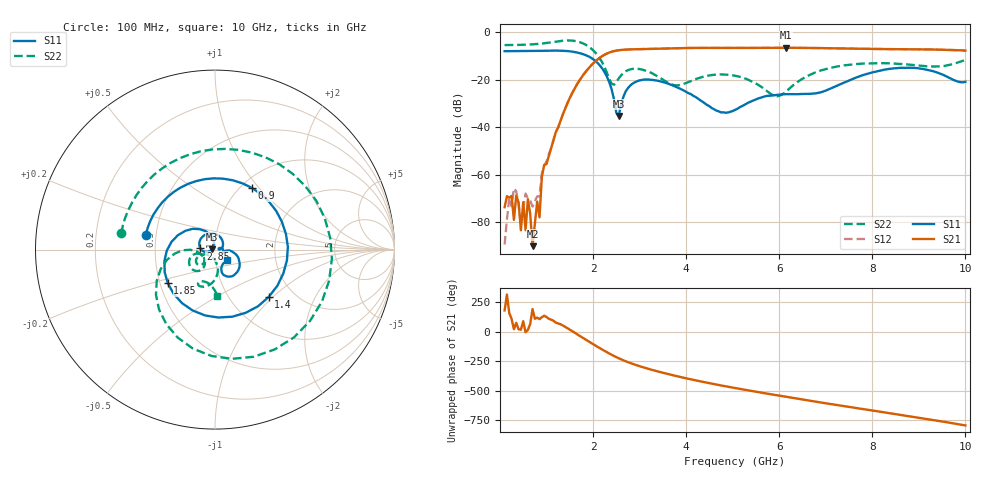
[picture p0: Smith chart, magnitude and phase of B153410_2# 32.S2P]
!  2-Port S-parameters saved by WinCal
! VAR MeasName=S-Parameters (CALIBRATED_DATA) read from VNA (N5245A)
! VAR MeasDate=2016-12-23 10:00:58
! VAR NAME=B153410_2# 32
! VAR FILENAME=B153410_2# 32.S2P
! VAR DATE=2016-12-23 10:00:58
! VAR PHYS_PORTS=1,2
# Hz S DB R 50
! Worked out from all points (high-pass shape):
!   199 points, 100 MHz to 10 GHz, reference 50 ohm
!   highest |S21| = -6.64 dB at 6.15 GHz (marker M1); lowest = -90.1 dB at 700 MHz (marker M2)
!   |S21| within 3 dB of the highest: 2.242 GHz to end of sweep
!   lowest |S11| = -35.4 dB at 2.55 GHz (marker M3), VSWR 1.03, Z = 48.3 + j0.252 ohm
!   |S11| at or under -10 dB: 1.871 GHz to end of sweep
!   |S22| runs from -27.1 to -3.6 dB; largest |S21 - S12| = 0.004
!   S11 on the Smith chart (normalised r, x): 100 MHz: 0.44, +0.08; 900 MHz: 1.12, +0.92; 1.4 GHz: 1.50, -0.94; 1.85 GHz: 0.55, -0.23; 2.85 GHz: 0.85, +0.01; 10 GHz: 1.13, -0.14
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1e8  -8.09 168.3  -73.70 179.7  -89.45 106.2  -5.52 170.2
2.5e8  -8.08 150.5  -68.95 108.5  -73.32 155.5  -5.50 155.4
3e8  -8.09 144.6  -79.04 21.0  -65.81 103.7  -5.50 150.2
3.5e8  -8.07 138.4  -68.80 74.9  -67.04 117.1  -5.47 145.1
4.5e8  -8.07 125.8  -83.41 16.8  -80.80 49.5  -5.42 134.3
6e8  -8.05 105.6  -70.33 15.2  -69.94 71.8  -5.31 117.2
7e8  -8.02 91.2  -90.08 -168.8  -73.45 45.7  -5.21 104.9
8e8  -7.99 75.8  -71.31 119.6  -69.12 111.3  -5.06 91.5
8.5e8  -7.97 67.7  -77.96 106.2  -69.22 146.3  -4.98 84.4
9e8  -7.95 59.3  -61.03 122.7  -59.40 134.3  -4.87 77.1
1.4e9  -7.98 -41.4  -32.26 41.6  -32.28 42.2  -3.62 -15.1
1.75e9  -9.11 -121.7  -19.19 -44.5  -19.18 -44.3  -4.54 -92.0
1.85e9  -9.82 -144.6  -16.55 -68.9  -16.53 -68.9  -5.47 -112.9
2.25e9  -16.99 126.5  -9.55 -162.9  -9.55 -163.0  -14.94 -178.9
2.55e9  -35.38 171.2  -7.69 135.7  -7.70 135.8  -19.59 -123.4
2.85e9  -21.71 175.5  -7.31 88.2  -7.29 88.2  -15.53 -138.4
3.4e9  -20.55 103.8  -7.01 23.1  -7.02 23.0  -18.83 -167.5
5.05e9  -32.77 18.8  -6.71 -116.4  -6.73 -116.3  -18.40 -151.5
6.15e9  -26.15 -12.6  -6.64 169.3  -6.66 169.4  -24.98 -93.2
6.7e9  -25.96 -13.9  -6.72 133.7  -6.74 133.7  -17.65 -83.7
8.35e9  -15.57 -35.0  -7.23 32.7  -7.21 33.0  -13.17 -114.5
1e10  -20.95 -42.3  -7.85 -72.8  -7.87 -72.5  -11.74 -87.2
